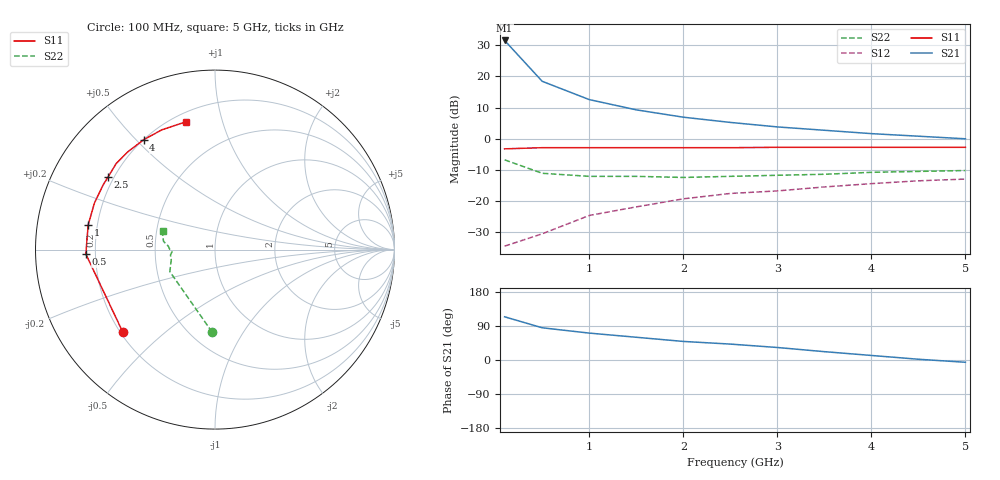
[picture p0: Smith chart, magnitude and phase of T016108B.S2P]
!AT-01610
!S-PARAMETERS at Vce=8V  Ic=60mA.  LAST UPDATED 07-21-92
!OBSOLETED Feb 1994 - nearest replacement: AT-42010
# ghz s ma r 50
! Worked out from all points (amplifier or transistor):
!   11 points, 100 MHz to 5 GHz, reference 50 ohm
!   highest |S21| = 31.5 dB at 100 MHz (marker M1)
!   |S21| within 3 dB of that: start of sweep to 191.6 MHz
!   unconditionally stable (mu >= 1): 424.1 MHz to end of sweep
!   at 500 MHz: K = 1.10, MAG = 22.5 dB, |S12| = -30.5 dB
!   at 2.5 GHz: K = 1.16, MAG = 8.9 dB, |S12| = -17.5 dB
!   at 5 GHz: K = 1.14, MAG = 4.2 dB, |S12| = -12.9 dB
!   S11 on the Smith chart (normalised r, x): 100 MHz: 0.21, -0.37; 500 MHz: 0.16, -0.02; 1 GHz: 0.16, +0.09; 2.5 GHz: 0.18, +0.30; 4 GHz: 0.20, +0.53; 5 GHz: 0.25, +0.76
0.1  0.69 -138.0  37.69 114.0  0.019 42.0  0.46 -92.0
0.5  0.72 -178.0  8.34 85.0  0.03 60.0  0.28 -154.0
1  0.72 169.0  4.25 71.0  0.059 59.0  0.25 -167.0
1.5  0.72 159.0  2.91 60.0  0.081 59.0  0.25 -173.0
2  0.72 150.0  2.22 49.0  0.109 52.0  0.24 -177.0
2.5  0.72 146.0  1.83 42.0  0.133 54.0  0.25 -179.0
3  0.73 139.0  1.55 33.0  0.146 49.0  0.26 176.0
3.5  0.73 132.0  1.37 22.0  0.169 44.0  0.27 174.0
4  0.73 123.0  1.21 12.0  0.191 37.0  0.29 171.0
4.5  0.73 114.0  1.1 2.0  0.212 30.0  0.3 166.0
5  0.73 103.0  1 -6.0  0.226 24.0  0.31 160.0
